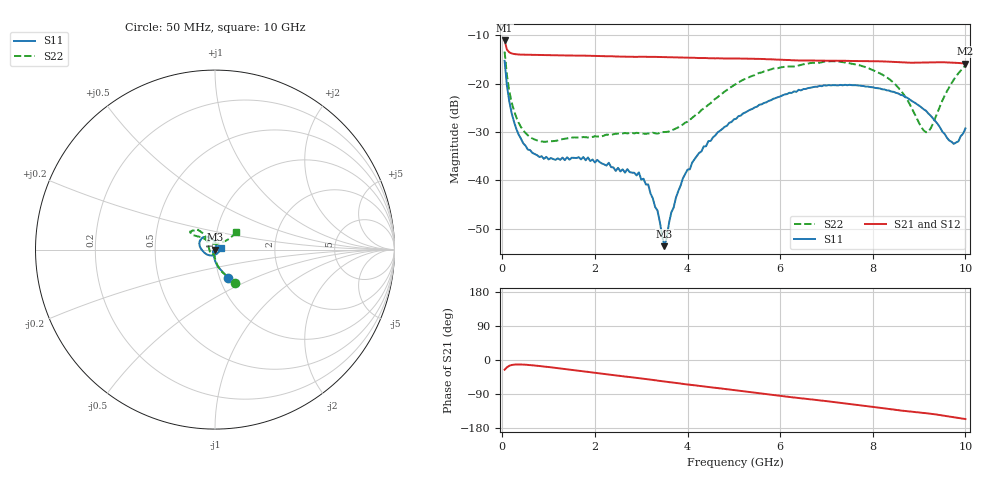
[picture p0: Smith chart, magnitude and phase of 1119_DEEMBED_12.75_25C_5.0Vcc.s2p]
!Hittite Microwave Corp.
!Digital Attenuator/PhaseShifter Rev 1.4.0
!Filename: C:\DATA\DATA\1119_DEEMBED_12.75_25C_5.0Vcc.s2p
!VNA ID: Agilent Technologies,N5224A,MY51441122,A.10.45.03
!Device type:
!2 Port Calibration.
!Temp(C): 25
!Lot Number:
!Serial Number:
!Operator:
!Misc:
!Attenuator:  12.750
# GHZ S DB R 50.0
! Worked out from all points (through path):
!   200 points, 50 MHz to 10 GHz, reference 50 ohm
!   highest |S21| = -11.03 dB at 50 MHz (marker M1); lowest = -15.8 dB at 10 GHz (marker M2)
!   group delay of S21, straight-line fit = 41.2 ps
!   lowest |S11| = -53.6 dB at 3.5 GHz (marker M3), VSWR 1.00, Z = 50.2 - j0.128 ohm
!   |S11| at or under -10 dB: start of sweep to end of sweep
!   |S22| runs from -32.0 to -13.3 dB; largest |S21 - S12| = 0.00066
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0.05  -15.24 -65.3  -11.03 -25.6  -11.03 -25.6  -13.34 -59.7
0.1  -20.38 -80.8  -12.93 -19.3  -12.92 -19.3  -18.24 -74.8
0.2  -25.97 -93.7  -13.71 -13.3  -13.71 -13.3  -23.74 -86.1
0.35  -30.46 -104.4  -13.93 -11.7  -13.93 -11.7  -28.00 -92.9
0.55  -33.60 -116.5  -14.01 -12.9  -14.00 -12.9  -30.64 -98.8
0.9  -35.54 -127.4  -14.06 -17.2  -14.07 -17.2  -31.99 -104.9
1.75  -35.15 -133.7  -14.17 -29.8  -14.18 -29.8  -31.02 -115.0
2.95  -38.33 -105.0  -14.40 -47.9  -14.41 -47.9  -30.21 -152.3
3.15  -40.82 -94.6  -14.42 -51.0  -14.43 -51.0  -30.28 -162.4
3.4  -48.47 -84.7  -14.44 -54.9  -14.45 -55.0  -30.16 -174.6
3.5  -53.60 -37.8  -14.45 -56.6  -14.45 -56.6  -29.98 179.5
3.65  -46.60 30.1  -14.50 -58.9  -14.51 -59.0  -29.67 171.8
4  -37.76 57.0  -14.60 -64.5  -14.61 -64.5  -27.85 151.8
4.45  -31.87 70.8  -14.71 -71.3  -14.72 -71.4  -24.34 134.7
5.05  -27.24 89.8  -14.78 -80.0  -14.79 -80.1  -20.01 126.6
6.7  -20.72 130.7  -15.17 -104.4  -15.18 -104.4  -15.66 139.8
7.65  -20.30 153.9  -15.28 -118.3  -15.29 -118.4  -16.02 147.0
8.35  -21.39 169.4  -15.42 -129.3  -15.42 -129.3  -18.98 140.6
8.65  -22.39 179.4  -15.56 -133.9  -15.55 -133.9  -21.94 133.6
9.15  -25.58 -148.6  -15.59 -140.3  -15.60 -140.3  -30.03 90.5
9.75  -32.44 -46.9  -15.64 -151.0  -15.65 -151.0  -19.12 37.4
10  -29.24 11.3  -15.80 -155.9  -15.81 -155.8  -16.21 39.4
